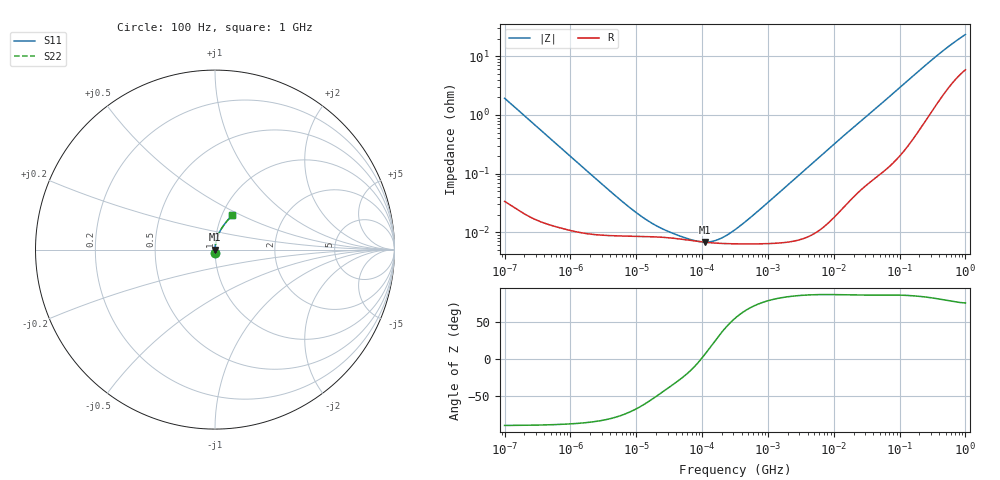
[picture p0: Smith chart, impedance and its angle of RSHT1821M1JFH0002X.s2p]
! RSHT1821M1JFH0002X  S-PARAMETER MODEL  (General Type)
! Model Generated by ELNA Corporation (http://www.ty-top.com)
! Version 1.0
! ELNA Control No.201028
! Copyright (c) 2020 ELNA CO.,LTD. All Rights Reserved.
! Products Name : CONDUCTIVE POLYMER HYBRID ALUMINUM ELECTROLYTIC CAPACITORS
! Characteristics :
!  Capacitance  :  820uF  ,  Rated voltage  :  6.3V
!  Operating Temp. Range  :  -55 to +105 degC  ,  Endurance  :  5000hr at 105 degC
!  Dimension D  :  10mm  ,  Dimension L  :  10mm
! Frequency Range : 100Hz - 1GHz
! External Node Assignments :
!  1  o---| |---o  2
# MHz S RI R 50
!Freq[MHz].  S11 Real  S11 Imag  S21 Real  S21 Imag  S12 Real  S12 Imag  S22 Real  S22 Imag
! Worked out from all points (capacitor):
!   401 points, 100 Hz to 1 GHz, reference 50 ohm
!   read as one part in series: C = 826 uF near 108 Hz
!   lowest |Z| = 6.79 mohm at 110.9 kHz (marker M1)
!   series resonance near 96.35 kHz, so ESL is about 3.3 nH
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0.0001  0.000704 -0.0192  0.9993 0.0192  0.9993 0.0192  0.000704 -0.0192
0.000133  0.000485 -0.0145  0.9995 0.0145  0.9995 0.0145  0.000485 -0.0145
0.001488  9.93e-05 -0.00132  0.9999 0.00132  0.9999 0.00132  9.93e-05 -0.00132
0.004597  8.72e-05 -0.000429  0.9999 0.000429  0.9999 0.000429  8.72e-05 -0.000429
0.008414  8.56e-05 -0.000235  0.9999 0.000235  0.9999 0.000235  8.56e-05 -0.000235
0.014207  8.44e-05 -0.00014  0.9999 0.00014  0.9999 0.00014  8.44e-05 -0.00014
0.022131  8.27e-05 -8.99e-05  0.9999 8.99e-05  0.9999 8.99e-05  8.27e-05 -8.99e-05
0.030549  8.05e-05 -6.44e-05  0.9999 6.44e-05  0.9999 6.44e-05  8.05e-05 -6.44e-05
0.034475  7.95e-05 -5.65e-05  0.9999 5.65e-05  0.9999 5.65e-05  7.95e-05 -5.65e-05
0.110917  6.74e-05 8.05e-06  0.9999 -8.05e-06  0.9999 -8.05e-06  6.74e-05 8.05e-06
0.258523  6.37e-05 6.97e-05  0.9999 -6.97e-05  0.9999 -6.97e-05  6.37e-05 6.97e-05
0.291743  6.35e-05 8.16e-05  0.9999 -8.16e-05  0.9999 -8.16e-05  6.35e-05 8.16e-05
0.316228  6.34e-05 9.02e-05  0.9999 -9.02e-05  0.9999 -9.02e-05  6.34e-05 9.02e-05
0.707946  6.34e-05 0.00022  0.9999 -0.00022  0.9999 -0.00022  6.34e-05 0.00022
4.704354  9.26e-05 0.00149  0.9999 -0.00149  0.9999 -0.00149  9.26e-05 0.00149
13.4122  0.000266 0.00417  0.9997 -0.00417  0.9997 -0.00417  0.000266 0.00417
69.9842  0.00173 0.0203  0.9983 -0.0203  0.9983 -0.0203  0.00173 0.0203
169.8244  0.00653 0.048  0.9935 -0.048  0.9935 -0.048  0.00653 0.048
365.1741  0.0243 0.096  0.9757 -0.096  0.9757 -0.096  0.0243 0.096
641.9482  0.0572 0.1471  0.9428 -0.1471  0.9428 -0.1471  0.0572 0.1471
922.5714  0.0888 0.1846  0.9112 -0.1846  0.9112 -0.1846  0.0888 0.1846
1000  0.0968 0.1936  0.9032 -0.1936  0.9032 -0.1936  0.0968 0.1936
